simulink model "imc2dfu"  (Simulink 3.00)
settings: Solver=ode45  SolverMode=SingleTasking  StartTime=0.0  StopTime=10  FixedStep=st_size  MaxStep=st_size  RelTol=1e-5  AbsTol=1e-6
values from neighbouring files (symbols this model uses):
  Disturb = Setpoint    [mimo_MSF1DF_sim.m]    (also in mimo_MSF2DF_sim.m)
  Satlb = temp1    [cback.m]    (also in imcmenu.m = str2num(satlbs))
  Satub = temp1    [cback.m]    (also in imcmenu.m = str2num(satubs))
  Setpoint = zeros(1,n)    [mimo_MSF1DF_sim.m]    (also in mimo_MSF2DF_sim.m)
undefined symbols (not defined in the file or in its folder): Csden, Csnum, denPs, numPs, Pdelay, Pre_fil_den, Pre_fil_num

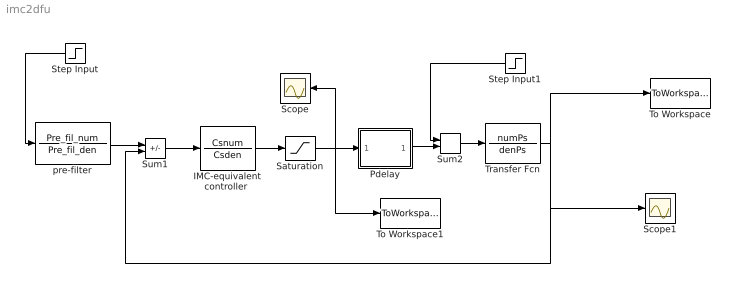
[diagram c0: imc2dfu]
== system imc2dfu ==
  "IMC-equivalent controller " : TransferFcn  Numerator=Csnum  Denominator=Csden
  Pdelay : Subsystem
  Saturation : Saturate  UpperLimit=Satub  LowerLimit=Satlb
  Scope : Scope
  Scope1 : Scope
  Step Input : Step  Orientation=left  Time=0  Before=0  After=Setpoint  SampleTime=0
  Step Input1 : Step  Orientation=left  Time=0  Before=0  After=Disturb  SampleTime=0
  Sum1 : Sum  Inputs=+-  SaturateOnIntegerOverflow=on
  Sum2 : Sum  Inputs=++  SaturateOnIntegerOverflow=on
  To Workspace : ToWorkspace  VariableName=simout  SampleTime=-1  SaveFormat=Matrix
  To Workspace1 : ToWorkspace  VariableName=effort  SampleTime=-1  SaveFormat=Matrix
  Transfer Fcn : TransferFcn  Numerator=numPs  Denominator=denPs
  pre-filter : TransferFcn  Numerator=Pre_fil_num  Denominator=Pre_fil_den
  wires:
  Sum1/1 -> "IMC-equivalent controller "/1
  Step Input/1 -> pre-filter/1
  "IMC-equivalent controller "/1 -> Saturation/1
  pre-filter/1 -> Sum1/1
  Step Input1/1 -> Sum2/1
  Pdelay/1(Out1) -> Sum2/2
  Sum2/1 -> Transfer Fcn/1
  Saturation/1 -> Pdelay/1(In1), To Workspace1/1, Scope/1
  Transfer Fcn/1 -> Sum1/2, To Workspace/1, Scope1/1

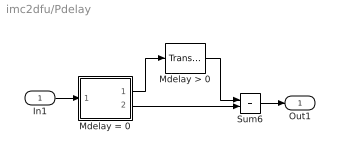
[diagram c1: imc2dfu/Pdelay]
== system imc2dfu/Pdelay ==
  In1 : Inport  Port=1  PortWidth=-1  SampleTime=-1  DataType=auto
  Mdelay > 0 : TransportDelay  DelayTime=Pdelay  InitialInput=0  BufferSize=1024
  Mdelay = 0 : Subsystem  Description=pass input signal through out1 if condition is true.
  Sum6 : Sum  Inputs=++  SaturateOnIntegerOverflow=on
  Out1 : Outport  Port=1
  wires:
  Mdelay = 0/1(Out2) -> Mdelay > 0/1
  Mdelay > 0/1 -> Sum6/1
  Mdelay = 0/2(Out1) -> Sum6/2
  In1/1 -> Mdelay = 0/1(In)
  Sum6/1 -> Out1/1

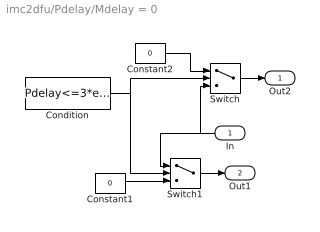
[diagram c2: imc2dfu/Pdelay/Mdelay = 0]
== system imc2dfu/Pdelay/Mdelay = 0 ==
  In : Inport  Orientation=left  Port=1  PortWidth=-1  SampleTime=-1  DataType=auto
  Condition : Constant  Value=Pdelay<=3*eps
  Constant1 : Constant  Value=0
  Constant2 : Constant  Value=0
  Switch : Switch  Threshold=1
  Switch1 : Switch  Threshold=1
  Out2 : Outport  Port=1  InitialOutput=0
  Out1 : Outport  Port=2  InitialOutput=0
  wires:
  In/1 -> Switch/3, Switch1/1
  Condition/1 -> Switch1/2, Switch/2
  Constant1/1 -> Switch1/3
  Constant2/1 -> Switch/1
  Switch/1 -> Out2/1
  Switch1/1 -> Out1/1
